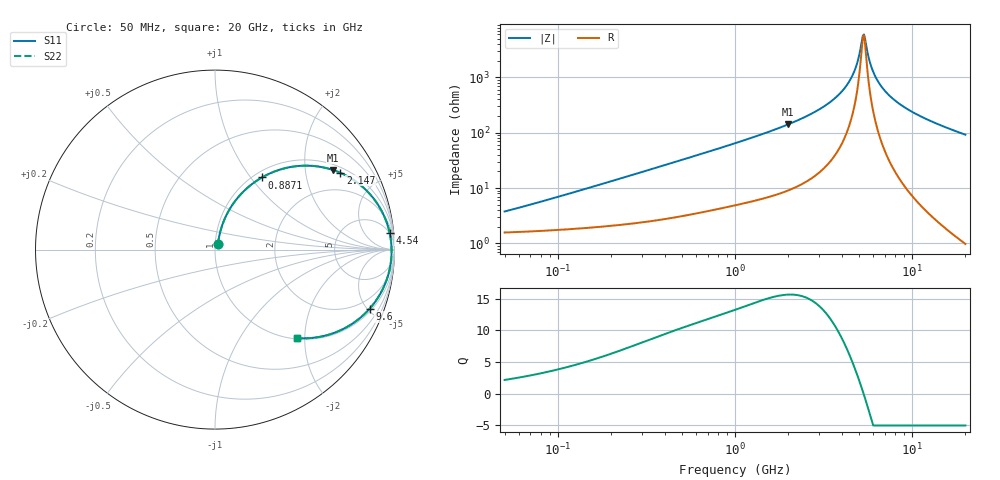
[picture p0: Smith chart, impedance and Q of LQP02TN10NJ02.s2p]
!Murata Part Number: LQP02TN10NJ02
!These Parameters are Measured in Series Mode Connection
!  o--[Z]--o
!Port1  Port2
!  o-------o
!Freq. Start=50[MHz] Stop=20[GHz], 401[Steps]
# Hz S RI R 50
!Freq.(Hz) S11(Real) S11(Imag) S21(Real) S21(Imag) S12(Real) S12(Imag) S22(Real) S22(Imag)
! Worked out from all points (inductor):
!   401 points, 50 MHz to 20 GHz, reference 50 ohm
!   read as one part in series: L = 10.7 nH near 73.81 MHz
!   highest Q = 15.6 at 1.992 GHz (marker M1), where L = 11.3 nH
!   self-resonance near 5.273 GHz
!   S11 on the Smith chart (normalised r, x): 50 MHz: 1.03, +0.07; 887.1 MHz: 1.09, +1.14; 2.147 GHz: 1.20, +3.12; 4.54 GHz: 5, +19; 9.6 GHz: 1.17, -5.15; 20 GHz: 1.02, -1.84
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5e7  0.0166 0.0331  0.9834 -0.0331  0.9834 -0.0331  0.0166 0.0331
1.364002e8  0.026 0.0865  0.974 -0.0865  0.974 -0.0865  0.026 0.0865
3.721004e8  0.0763 0.2161  0.9237 -0.2161  0.9237 -0.2161  0.0763 0.2161
8.870719e8  0.2615 0.4019  0.7385 -0.4019  0.7385 -0.4019  0.2615 0.4019
1e9  0.307 0.425  0.693 -0.425  0.693 -0.425  0.307 0.425
1.99176e9  0.6567 0.4439  0.3433 -0.4439  0.3433 -0.4439  0.6567 0.4439
2.146657e9  0.6976 0.4284  0.3024 -0.4284  0.3024 -0.4284  0.6976 0.4284
2.728004e9  0.8182 0.3531  0.1818 -0.3531  0.1818 -0.3531  0.8182 0.3531
3.736399e9  0.9339 0.2048  0.0661 -0.2048  0.0661 -0.2048  0.9339 0.2048
4.149438e9  0.9582 0.1468  0.0418 -0.1468  0.0418 -0.1468  0.9582 0.1468
4.539627e9  0.9727 0.0949  0.0273 -0.0949  0.0273 -0.0949  0.9727 0.0949
4.89267e9  0.9803 0.0506  0.0197 -0.0506  0.0197 -0.0506  0.9803 0.0506
5.194772e9  0.9834 0.0148  0.0166 -0.0148  0.0166 -0.0148  0.9834 0.0148
5.352748e9  0.9839 -0.00324  0.0161 0.00324  0.0161 0.00324  0.9839 -0.00324
5.433528e9  0.9839 -0.0122  0.0161 0.0122  0.0161 0.0122  0.9839 -0.0122
5.856089e9  0.9814 -0.0573  0.0186 0.0573  0.0186 0.0573  0.9814 -0.0573
6.125241e9  0.9778 -0.0842  0.0222 0.0842  0.0222 0.0842  0.9778 -0.0842
6.701223e9  0.9662 -0.1374  0.0338 0.1374  0.0338 0.1374  0.9662 -0.1374
7.442007e9  0.945 -0.1977  0.055 0.1977  0.055 0.1977  0.945 -0.1977
9.600142e9  0.8609 -0.33  0.1391 0.33  0.1391 0.33  0.8609 -0.33
1.396067e10  0.6703 -0.4617  0.3297 0.4617  0.3297 0.4617  0.6703 -0.4617
2e10  0.4594 -0.4931  0.5406 0.4931  0.5406 0.4931  0.4594 -0.4931
